(* Logix 5000 AddOnInstructionDefinition export HI6200_Faceplate_AOI; software revision 30.00 *)

ADD_ON_INSTRUCTION HI6200_Faceplate_AOI   (* revision 1.1, vendor Hardy Process Solutions *)
// AOI to run sample faceplate.
// Revision note:
// modified tag names to be more descriptive.
// Made code more efficient.
VAR_OUTPUT
   cal_status : SINT; {access Read Only}   // filtered cal status
END_VAR
VAR_INPUT
   fp_dis_md : INT;   // weight select
END_VAR
VAR_OUTPUT
   cmd_status : DINT; {access Read Only}   // filtered cmd status
END_VAR
VAR_IN_OUT
   Input_hi6200 : _0102:Hardy6200Series_F6857DC7:I:0; {required}
   Output_hi6200 : _0102:Hardy6200Series_52E4DDE0:O:0; {required}
END_VAR
VAR_INPUT
   pm_2881 : DINT;   // Units of measure
END_VAR
VAR_OUTPUT
   hardy_6200_inst_st : INT; {access Read Only}   // Instrument Status
   hardy_6200_net_wt : REAL; {access Read Only}   // Net Weight
   hardy_6200_gross_wt : REAL; {access Read Only}   // Gross weight
END_VAR
VAR_INPUT
   pm_4101 : REAL;   // Ref Weight
   pm_4182 : REAL;   // Span Weight
   pm_4102 : REAL;   // Gravity Correction
   pm_2081 : DINT;   // WAVERSAVER
   pm_2082 : DINT;   // Averages
   pm_6301 : DINT;   // Auto Zero Tracking Enable
   reset_az_enable_indication : BOOL;   // reset pointer on HMI list for Zero Tracking
   pm_6302 : REAL;   // Auto Zero tolerance
   pm_2886 : REAL;   // Zero Tolerance
END_VAR
VAR_OUTPUT
   pm_6201 : REAL;   // previous zerod amount
END_VAR
VAR_INPUT
   reset_units_indication : BOOL;   // reset pointer on HMI list for units of measure
   pm_2887 : REAL;   // Motion tolerance
   pm_6183 : REAL;   // Tare Weight
   reset_waversaver_indicator : BOOL;   // reset pointer on HMI list for WAVERSAVER
   rd_filter_settings : BOOL;   // Read filter settings
   input_cmd_status : INT;   // Filtered Cmd Status
   rd_zero_tare_settings : BOOL;   // read zero and tare settings
   rd_setup1_settings : BOOL;   // read setup 1 settings
   rd_c2cal_settings : BOOL;   // read C2 cal settings
   rd_tradcal_settings : BOOL;   // program control bit to read hard cal ref weight
   zero_cmd : BOOL;   // trigger zero command
   tare_cmd : BOOL;   // trigger tare command
   cal_low_cmd : BOOL;   // Cal Low trigger
   cal_high_cmd : BOOL;   // Cal High trigger
   c2_cmd : BOOL;   // C2 cal trigger
   write_C2_cal_settings : BOOL;   // trigger write C2 settings
   write_tradcal_settings : BOOL;   // trigger write hard cal settings
   write_filter_settings : BOOL;   // trigger write filter settings
   write_zero_tare_settings : BOOL;   // trigger write zero and tare settings
   write_units_setting : BOOL;   // trigger write units of measure
   pm_2888 : REAL;   // Capacity
   rd_setup2_settings : BOOL;   // read setup 2 settings
   pm_2882 : DINT;   // Decimal places
   pm_2883 : DINT;   // Grad size
   reset_decimalpoint_indication : BOOL;   // reset pointer on HMI list for decimal point
   reset_grads_indication : BOOL;   // reset pointer on HMI list for grad size
   pm_4081 : DINT;   // Sensitivity
   reset_sensitivity_indication : BOOL;   // reset pointer on HMI list for sensitivity
   write_setup2_settings : BOOL;   // trigger write ins settup 2 settings
   write_setup1_settings : BOOL;   // trigger write ins setup 1 settings
END_VAR
VAR_IN_OUT
   config_6200 : _0102:Hardy6200Series_ABC98FB2:C:0; {required}
END_VAR
VAR_INPUT
   percent_weight : REAL;   // percent of full scale for trend
   Set_FaceplateAnimation : INT;   // HMI panel control
   pm_2081w : DINT;   // write value setting for WAVERSAVER
   pm_6301w : DINT;   // write value setting for auto zero tracking enable
   pm_2881w : DINT;   // write value for setting units of measure
   pm_2882w : DINT;   // write value for setting decimal places
   pm_2883w : DINT;   // write value for setting grad size
   pm_4081w : DINT;   // write value for setting sensitivity value
END_VAR
VAR
   initial_unit_rd : BOOL; {access None}   // program control bit to initial read of units of measure
   cmd_no : INT; {access None}   // cmd num holding register
   ons_1 : BOOL; {access None}
   ons_2 : BOOL; {access None}
   rd_waversaver : BOOL; {access None}   // read WAVERSAVER setting
   delay_reset_waversaer_ind : TIMER := (PRE := 200); {access None}   // operational delay timer
   rd_az_zero_tol : BOOL; {access None}   // read auto zero tolerance
   delay_reset_az_enable_indication : TIMER := (PRE := 200); {access None}   // operational delay timer
   rd_zero_tol : BOOL; {access None}   // read zero tolerance
   rd_zero_amount : BOOL; {access None}   // read zero'd amount
   ons_3 : BOOL; {access None}
   rd_motion_tol : BOOL; {access None}   // program control for read motion tol
   rd_capacity : BOOL; {access None}   // program control for read capacity
   delay_reset_units_indication : TIMER := (PRE := 200); {access None}   // operational delay timer
   ons_4 : BOOL; {access None}
   rd_c2cal_ref_wt : BOOL; {access None}   // program control during read C2 cal ref weight
   ons_5 : BOOL; {access None}
   rd_tradcal_span_wt : BOOL; {access None}   // program control bit to read hard cal span weight
   ons_6 : BOOL; {access None}
   ons_7 : BOOL; {access None}
   ons_8 : BOOL; {access None}
   ons_9 : BOOL; {access None}
   ons_10 : BOOL; {access None}
   run_cmd : BOOL; {access None}   // program control bit
   run_cmd_delay : TIMER := (PRE := 1000); {access None}   // Delay timer to allow time for process to complete
   ons_11 : BOOL; {access None}
   wr_C2_ref_wt : BOOL; {access None}   // program control bit writing C2 ref weight
   chec_status_wr_C2_ref : BOOL; {access None}   // operational code control bit writing C2 ref
   wr_gravity_correction : BOOL; {access None}   // program control bit writing gravity correction
   check_status_wr_gravity_correction : BOOL; {access None}   // operational code control bit write gravity correction
   ons_12 : BOOL; {access None}
   wr_hard_cal_ref_wt : BOOL; {access None}   // program control bit writing hard cal ref weight
   check_status_wr_traditional_ref : BOOL; {access None}   // operational code control bit write hard cal ref
   wr_span_wt : BOOL; {access None}   // program control bit writing span weight
   check_status_wr_span_wt : BOOL; {access None}   // operational code control bit write span weight
   ons_13 : BOOL; {access None}
   wr_waversaver : BOOL; {access None}   // program control bit writing WAVERSAVER
   check_status_wr_waversaver : BOOL; {access None}   // operational code control bit write WAVERSAVER
   wr_avgerages : BOOL; {access None}   // program control bit writing averages
   check_status_wr_averages : BOOL; {access None}   // operational code control bit write Averages
   wr_auto_zero_enable : BOOL; {access None}   // program control bit writing zuto zero enable
   check_status_wr_auto_zero_enable : BOOL; {access None}   // operational code control bit writing Auto Zero enable
   ons_14 : BOOL; {access None}
   wr_auto_zero_tolerance : BOOL; {access None}   // program control bit writing auto zero tolerance
   check_status_wr_auto_zero_tolerance : BOOL; {access None}   // operational code control bit writing Auto Zero tolerance
   wr_zero_tolerance : BOOL; {access None}   // program control bit writing zero tolerance
   check_status_wr_zero_tolerance : BOOL; {access None}   // operational code control bit write zero tolerance
   wr_units_measure : BOOL; {access None}   // program control bit writing units of measure
   ons_15 : BOOL; {access None}
   check_status_wr_units_measure : BOOL; {access None}   // operational code control bit write units of measure
   wr_motion_tolerance : BOOL; {access None}   // program control bit writing motion tolerance
   check_status_wr_motion_tolerance : BOOL; {access None}   // operational code control bit write motion tolerance
   wr_tare_weight : BOOL; {access None}   // program control bit writing tare weight
   check_status_wr_tare_weight : BOOL; {access None}   // operational code control bit write tare weight
   rd_tare_weight : BOOL; {access None}   // read tare weight
   ons_16 : BOOL; {access None}
   rd_grad_size : BOOL; {access None}   // program control bit for read grad size
   delay_reset_decimalpoint_indication : TIMER := (PRE := 200); {access None}   // operational delay timer
   delay_reset_grads_indication : TIMER := (PRE := 200); {access None}   // operational delay timer
   rd_hardcal_sensitivity : BOOL; {access None}   // program control bit to read hard cal sensitivity
   delay_reset_sensitivity_indication : TIMER := (PRE := 200); {access None}   // operational delay timer
   wr_sensitivity : BOOL; {access None}   // program control bit writing sensitivity
   check_status_wr_sensitivity : BOOL; {access None}   // operational code control bit write sensitivity
   wr_scale_capacity : BOOL; {access None}   // program control bit writing scale capacity
   check_status_wr_scale_capacity : BOOL; {access None}   // operational code control bit write scale capacity
   ons_17 : BOOL; {access None}
   wr_decimal_point : BOOL; {access None}   // program control bit writing decimal point
   check_status_wr_decimal_point : BOOL; {access None}   // operational code control bit writing decimal points
   wr_grad_size : BOOL; {access None}   // program control bit writing grad size
   check_status_wr_grads_size : BOOL; {access None}   // operational code control bit write grad size
   ons_18 : BOOL; {access None}
   rd_averages : BOOL; {access None}   // program control tag to read averages
   rd_autozero_state : BOOL; {access None}   // program control bit to read auto zero tracking state
   rd_units_measure : BOOL; {access None}   // program control bit to read the units of measure
   rd_decimal_places : BOOL; {access None}   // program control bit to read decima places
   rd_gravity : BOOL; {access None}   // program control bit to read gravity correction
   rd_traditional_cal_ref_wt : BOOL; {access None}   // program control bit to read traditional cal ref weight
   initial_capacity_rd : BOOL; {access None}   // program control bit to initial read of scale capacity
   initial_unit_rd_1 : BOOL; {access None}   // program control bit
   delay_dec_rd : TIMER := (PRE := 300); {access None}   // delay timer for decimal pt read
   delay_units_rd : TIMER := (PRE := 200); {access None}   // delay timer for units read
   delay_zstate_rd : TIMER := (PRE := 200); {access None}   // delay timer for zero state read
   delay_wave_rd : TIMER := (PRE := 200); {access None}   // delay timer for waversaver read
END_VAR

ROUTINE Logic   (* ladder *)
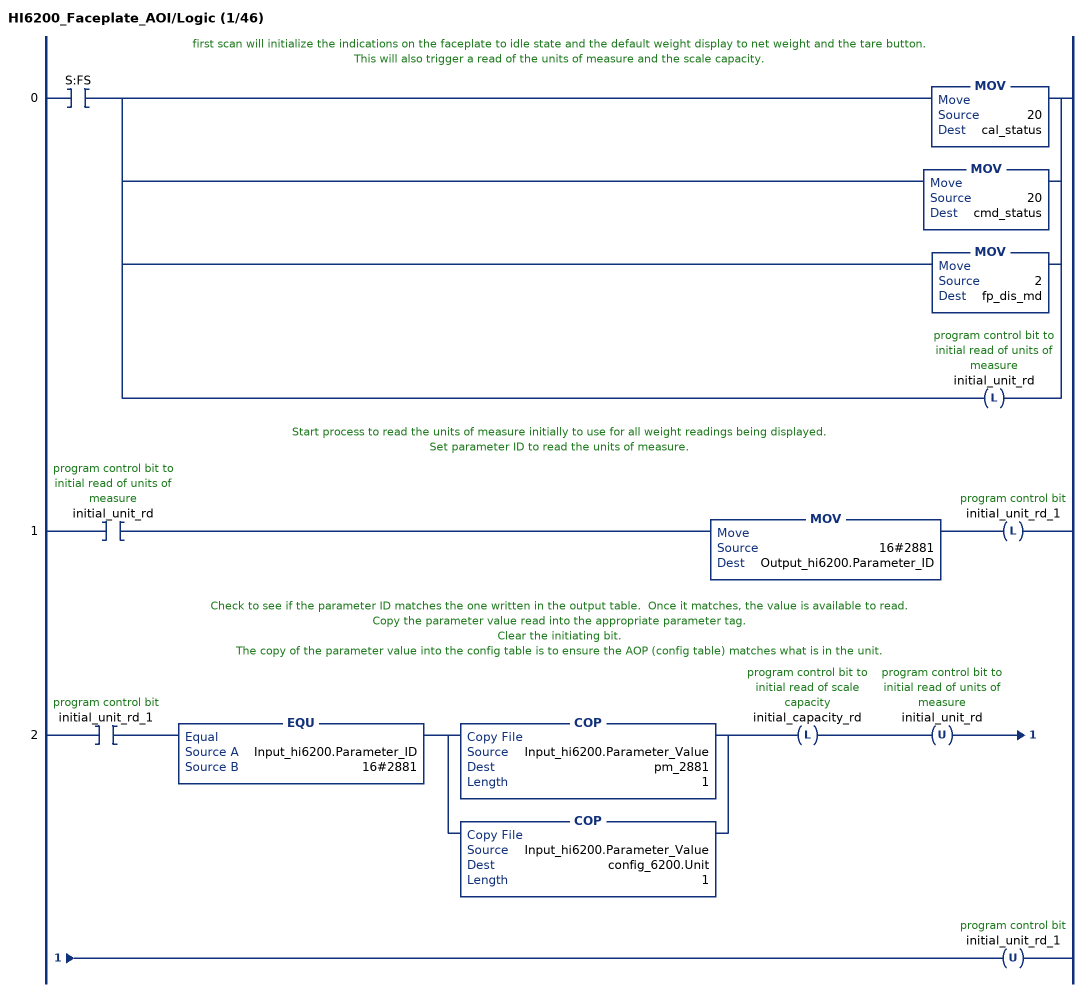
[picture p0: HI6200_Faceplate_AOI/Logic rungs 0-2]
   // first scan will initialize the indications on the faceplate to idle state and the default weight display to net weight and the tare button.
   // This will also trigger a read of the units of measure and the scale capacity.
   0: XIC(S:FS)[MOV(20,cal_status) ,MOV(20,cmd_status) ,MOV(2,fp_dis_md) ,OTL(initial_unit_rd) ];
   // Start process to read the units of measure initially to use for all weight readings being displayed.
   // Set parameter ID to read the units of measure.
   1: XIC(initial_unit_rd)MOV(16#2881,Output_hi6200.Parameter_ID)OTL(initial_unit_rd_1);
   // Check to see if the parameter ID matches the one written in the output table.  Once it matches, the value is available to read.
   // Copy the parameter value read into the appropriate parameter tag.
   // Clear the initiating bit.
   // The copy of the parameter value into the config table is to ensure the AOP (config table) matches what is in the unit.
   2: XIC(initial_unit_rd_1)EQU(Input_hi6200.Parameter_ID,16#2881)[COP(Input_hi6200.Parameter_Value,pm_2881,1) ,COP(Input_hi6200.Parameter_Value,config_6200.Unit,1) ]OTL(initial_capacity_rd)OTU(initial_unit_rd)OTU(initial_unit_rd_1);
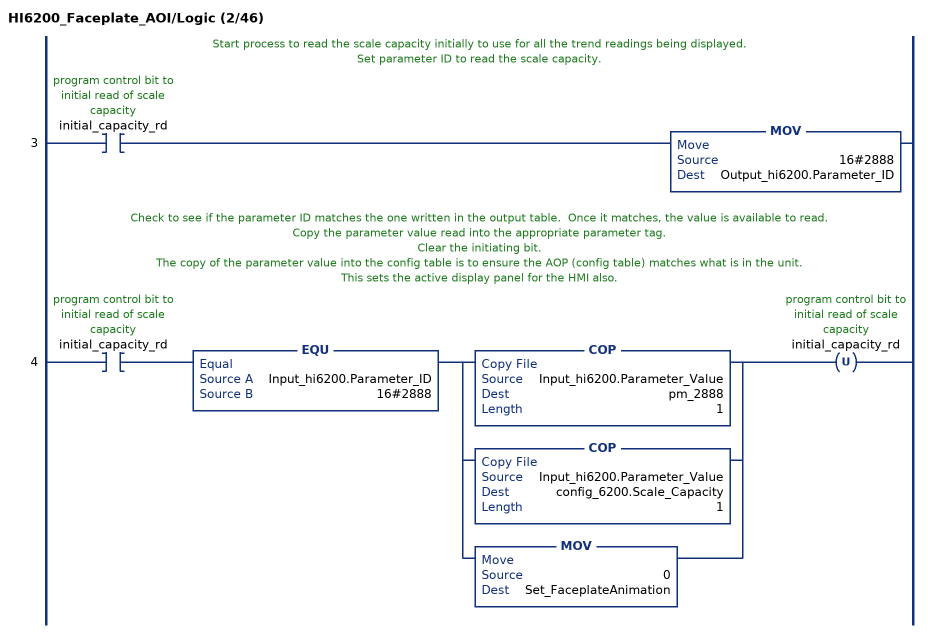
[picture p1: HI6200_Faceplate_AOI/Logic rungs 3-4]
   // Start process to read the scale capacity initially to use for all the trend readings being displayed.
   // Set parameter ID to read the scale capacity.
   3: XIC(initial_capacity_rd)MOV(16#2888,Output_hi6200.Parameter_ID);
   // Check to see if the parameter ID matches the one written in the output table.  Once it matches, the value is available to read.
   // Copy the parameter value read into the appropriate parameter tag.
   // Clear the initiating bit.
   // The copy of the parameter value into the config table is to ensure the AOP (config table) matches what is in the unit.
   // This sets the active display panel for the HMI also.
   4: XIC(initial_capacity_rd)EQU(Input_hi6200.Parameter_ID,16#2888)[COP(Input_hi6200.Parameter_Value,pm_2888,1) ,COP(Input_hi6200.Parameter_Value,config_6200.Scale_Capacity,1) ,MOV(0,Set_FaceplateAnimation) ]OTU(initial_capacity_rd);
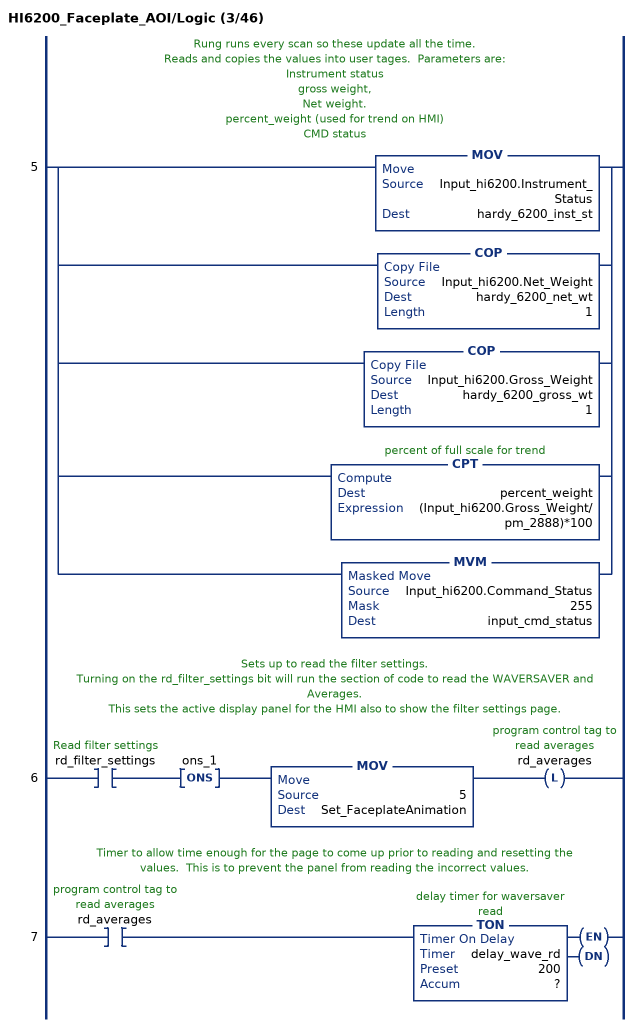
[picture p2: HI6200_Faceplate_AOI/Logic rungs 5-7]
   // Rung runs every scan so these update all the time.
   // Reads and copies the values into user tages.  Parameters are:
   // Instrument status
   // gross weight,
   // Net weight.
   // percent_weight (used for trend on HMI)
   // CMD status
   5: [MOV(Input_hi6200.Instrument_Status,hardy_6200_inst_st) ,COP(Input_hi6200.Net_Weight,hardy_6200_net_wt,1) ,COP(Input_hi6200.Gross_Weight,hardy_6200_gross_wt,1) ,CPT(percent_weight,(Input_hi6200.Gross_Weight/pm_2888)*100) ,MVM(Input_hi6200.Command_Status,255,input_cmd_status) ];
   // Sets up to read the filter settings.
   // Turning on the rd_filter_settings bit will run the section of code to read the WAVERSAVER and Averages.
   // This sets the active display panel for the HMI also to show the filter settings page.
   6: XIC(rd_filter_settings)ONS(ons_1)MOV(5,Set_FaceplateAnimation)OTL(rd_averages);
   // Timer to allow time enough for the page to come up prior to reading and resetting the values.  This is to prevent the panel from reading the incorrect values.
   7: XIC(rd_averages)TON(delay_wave_rd,?,?);
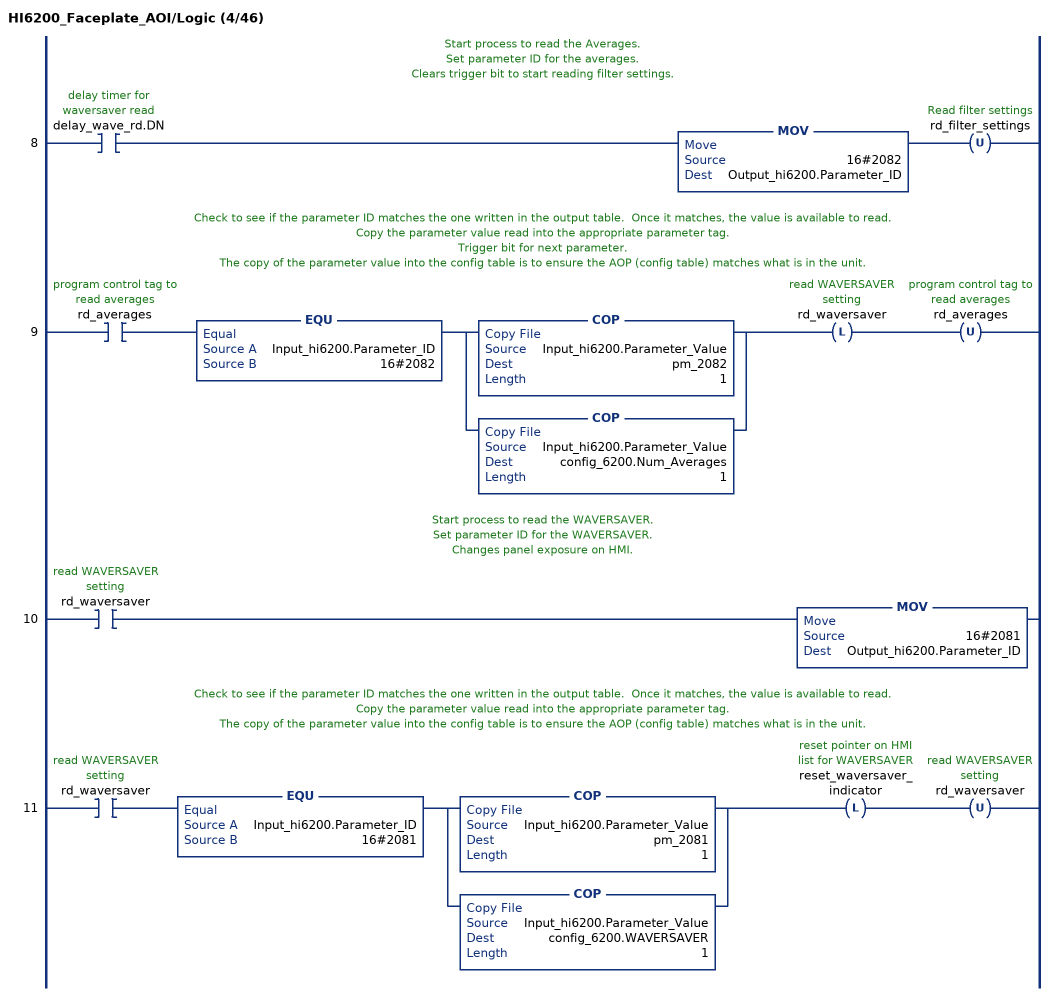
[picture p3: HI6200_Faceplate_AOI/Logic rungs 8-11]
   // Start process to read the Averages.
   // Set parameter ID for the averages.
   // Clears trigger bit to start reading filter settings.
   8: XIC(delay_wave_rd.DN)MOV(16#2082,Output_hi6200.Parameter_ID)OTU(rd_filter_settings);
   // Check to see if the parameter ID matches the one written in the output table.  Once it matches, the value is available to read.
   // Copy the parameter value read into the appropriate parameter tag.
   // Trigger bit for next parameter.
   // The copy of the parameter value into the config table is to ensure the AOP (config table) matches what is in the unit.
   9: XIC(rd_averages)EQU(Input_hi6200.Parameter_ID,16#2082)[COP(Input_hi6200.Parameter_Value,pm_2082,1) ,COP(Input_hi6200.Parameter_Value,config_6200.Num_Averages,1) ]OTL(rd_waversaver)OTU(rd_averages);
   // Start process to read the WAVERSAVER.
   // Set parameter ID for the WAVERSAVER.
   // Changes panel exposure on HMI.
   10: XIC(rd_waversaver)MOV(16#2081,Output_hi6200.Parameter_ID);
   // Check to see if the parameter ID matches the one written in the output table.  Once it matches, the value is available to read.
   // Copy the parameter value read into the appropriate parameter tag.
   // The copy of the parameter value into the config table is to ensure the AOP (config table) matches what is in the unit.
   11: XIC(rd_waversaver)EQU(Input_hi6200.Parameter_ID,16#2081)[COP(Input_hi6200.Parameter_Value,pm_2081,1) ,COP(Input_hi6200.Parameter_Value,config_6200.WAVERSAVER,1) ]OTL(reset_waversaver_indicator)OTU(rd_waversaver);
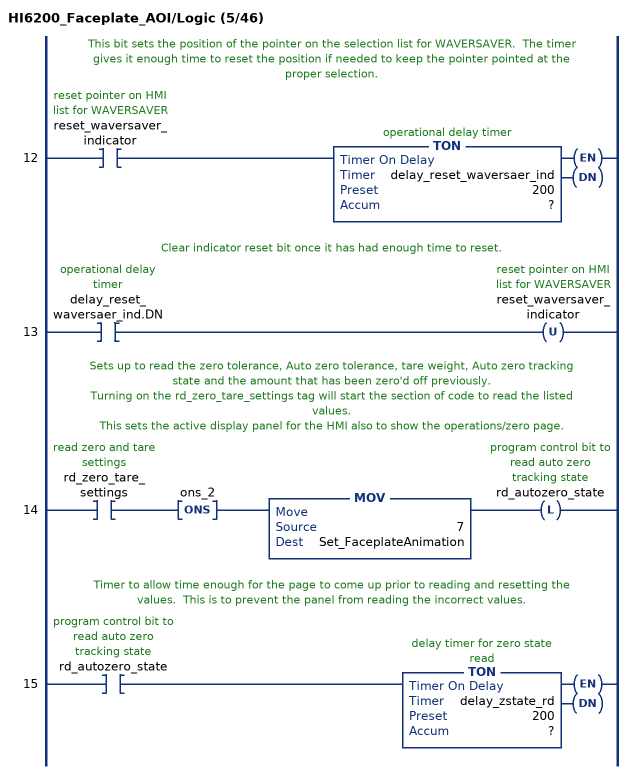
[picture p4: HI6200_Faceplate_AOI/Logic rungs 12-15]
   // This bit sets the position of the pointer on the selection list for WAVERSAVER.  The timer gives it enough time to reset the position if needed to keep the pointer pointed at the proper selection.
   12: XIC(reset_waversaver_indicator)TON(delay_reset_waversaer_ind,?,?);
   // Clear indicator reset bit once it has had enough time to reset.
   13: XIC(delay_reset_waversaer_ind.DN)OTU(reset_waversaver_indicator);
   // Sets up to read the zero tolerance, Auto zero tolerance, tare weight, Auto zero tracking state and the amount that has been zero'd off previously.
   // Turning on the rd_zero_tare_settings tag will start the section of code to read the listed values.
   // This sets the active display panel for the HMI also to show the operations/zero page.
   14: XIC(rd_zero_tare_settings)ONS(ons_2)MOV(7,Set_FaceplateAnimation)OTL(rd_autozero_state);
   // Timer to allow time enough for the page to come up prior to reading and resetting the values.  This is to prevent the panel from reading the incorrect values.
   15: XIC(rd_autozero_state)TON(delay_zstate_rd,?,?);
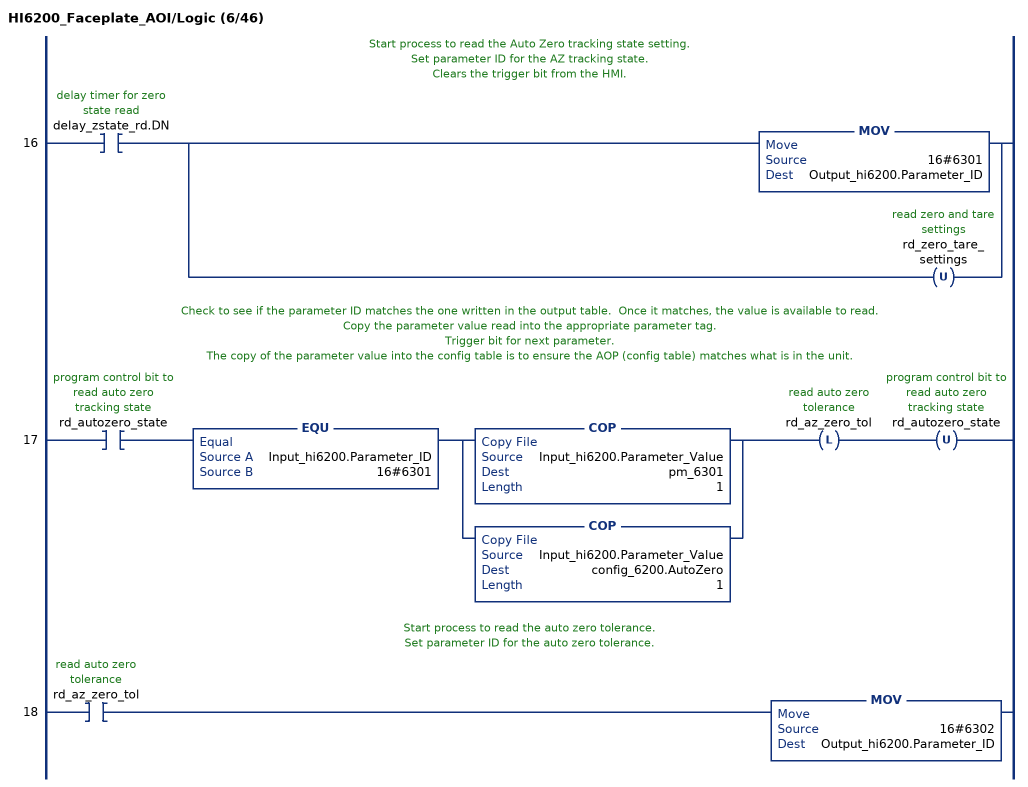
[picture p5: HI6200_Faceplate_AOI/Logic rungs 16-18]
   // Start process to read the Auto Zero tracking state setting.
   // Set parameter ID for the AZ tracking state.
   // Clears the trigger bit from the HMI.
   16: XIC(delay_zstate_rd.DN)[MOV(16#6301,Output_hi6200.Parameter_ID) ,OTU(rd_zero_tare_settings) ];
   // Check to see if the parameter ID matches the one written in the output table.  Once it matches, the value is available to read.
   // Copy the parameter value read into the appropriate parameter tag.
   // Trigger bit for next parameter.
   // The copy of the parameter value into the config table is to ensure the AOP (config table) matches what is in the unit.
   17: XIC(rd_autozero_state)EQU(Input_hi6200.Parameter_ID,16#6301)[COP(Input_hi6200.Parameter_Value,pm_6301,1) ,COP(Input_hi6200.Parameter_Value,config_6200.AutoZero,1) ]OTL(rd_az_zero_tol)OTU(rd_autozero_state);
   // Start process to read the auto zero tolerance.
   // Set parameter ID for the auto zero tolerance.
   18: XIC(rd_az_zero_tol)MOV(16#6302,Output_hi6200.Parameter_ID);
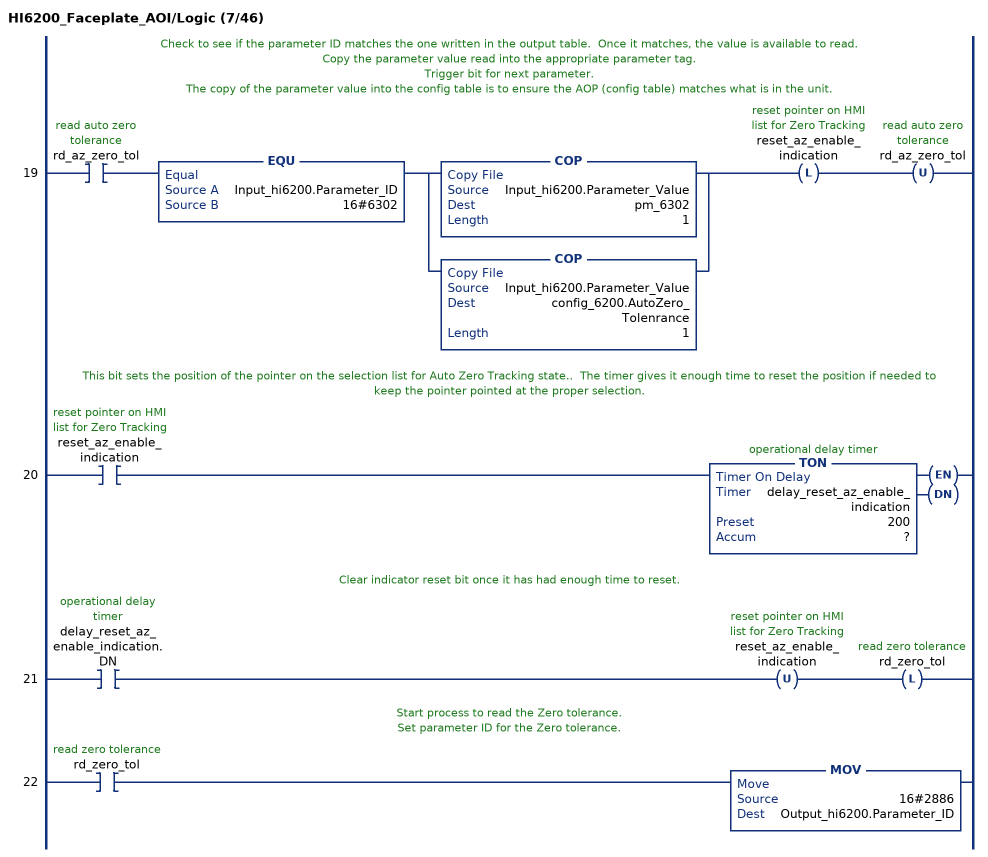
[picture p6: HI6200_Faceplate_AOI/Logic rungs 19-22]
   // Check to see if the parameter ID matches the one written in the output table.  Once it matches, the value is available to read.
   // Copy the parameter value read into the appropriate parameter tag.
   // Trigger bit for next parameter.
   // The copy of the parameter value into the config table is to ensure the AOP (config table) matches what is in the unit.
   19: XIC(rd_az_zero_tol)EQU(Input_hi6200.Parameter_ID,16#6302)[COP(Input_hi6200.Parameter_Value,pm_6302,1) ,COP(Input_hi6200.Parameter_Value,config_6200.AutoZero_Tolenrance,1) ]OTL(reset_az_enable_indication)OTU(rd_az_zero_tol);
   // This bit sets the position of the pointer on the selection list for Auto Zero Tracking state..  The timer gives it enough time to reset the position if needed to keep the pointer pointed at the proper selection.
   20: XIC(reset_az_enable_indication)TON(delay_reset_az_enable_indication,?,?);
   // Clear indicator reset bit once it has had enough time to reset.
   21: XIC(delay_reset_az_enable_indication.DN)OTU(reset_az_enable_indication)OTL(rd_zero_tol);
   // Start process to read the Zero tolerance.
   // Set parameter ID for the Zero tolerance.
   22: XIC(rd_zero_tol)MOV(16#2886,Output_hi6200.Parameter_ID);
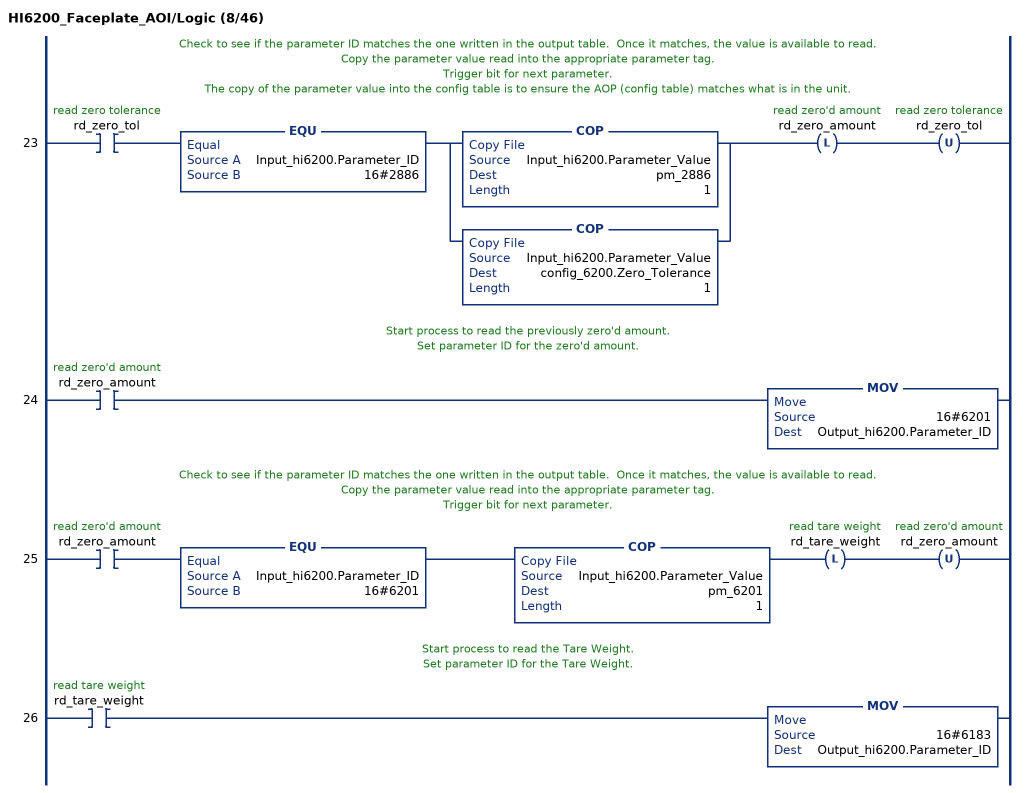
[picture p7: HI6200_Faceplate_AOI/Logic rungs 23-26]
   // Check to see if the parameter ID matches the one written in the output table.  Once it matches, the value is available to read.
   // Copy the parameter value read into the appropriate parameter tag.
   // Trigger bit for next parameter.
   // The copy of the parameter value into the config table is to ensure the AOP (config table) matches what is in the unit.
   23: XIC(rd_zero_tol)EQU(Input_hi6200.Parameter_ID,16#2886)[COP(Input_hi6200.Parameter_Value,pm_2886,1) ,COP(Input_hi6200.Parameter_Value,config_6200.Zero_Tolerance,1) ]OTL(rd_zero_amount)OTU(rd_zero_tol);
   // Start process to read the previously zero'd amount.
   // Set parameter ID for the zero'd amount.
   24: XIC(rd_zero_amount)MOV(16#6201,Output_hi6200.Parameter_ID);
   // Check to see if the parameter ID matches the one written in the output table.  Once it matches, the value is available to read.
   // Copy the parameter value read into the appropriate parameter tag.
   // Trigger bit for next parameter.
   25: XIC(rd_zero_amount)EQU(Input_hi6200.Parameter_ID,16#6201)COP(Input_hi6200.Parameter_Value,pm_6201,1)OTL(rd_tare_weight)OTU(rd_zero_amount);
   // Start process to read the Tare Weight.
   // Set parameter ID for the Tare Weight.
   26: XIC(rd_tare_weight)MOV(16#6183,Output_hi6200.Parameter_ID);
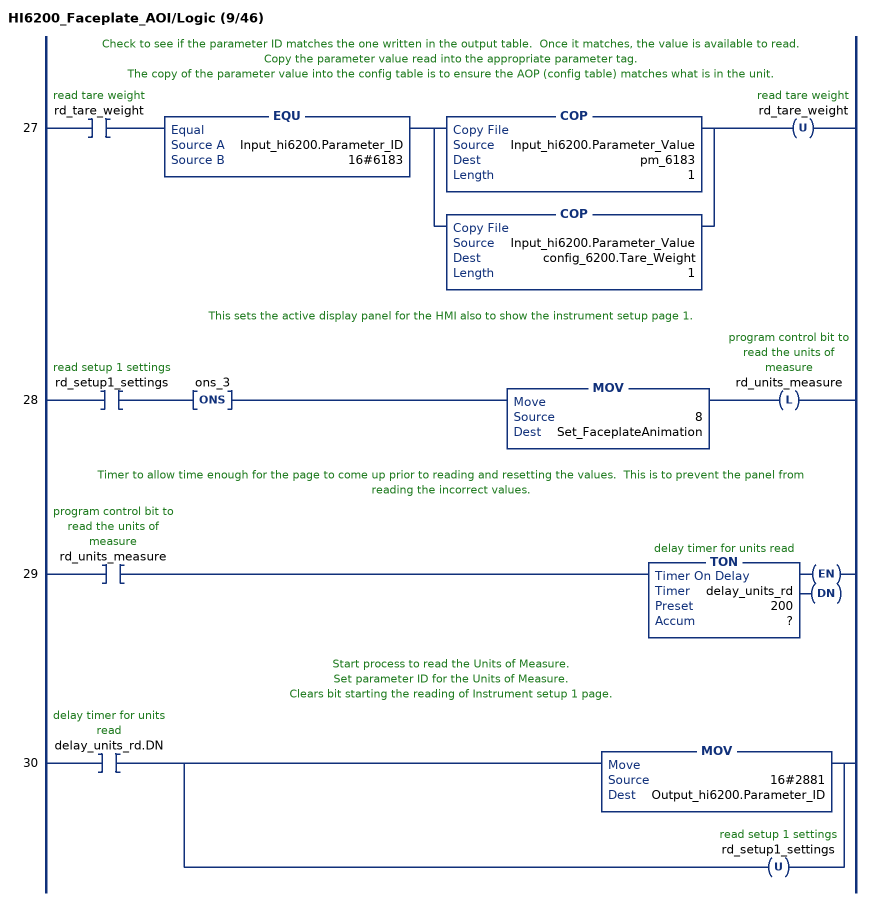
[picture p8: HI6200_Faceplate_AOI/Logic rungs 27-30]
   // Check to see if the parameter ID matches the one written in the output table.  Once it matches, the value is available to read.
   // Copy the parameter value read into the appropriate parameter tag.
   // The copy of the parameter value into the config table is to ensure the AOP (config table) matches what is in the unit.
   27: XIC(rd_tare_weight)EQU(Input_hi6200.Parameter_ID,16#6183)[COP(Input_hi6200.Parameter_Value,pm_6183,1) ,COP(Input_hi6200.Parameter_Value,config_6200.Tare_Weight,1) ]OTU(rd_tare_weight);
   // This sets the active display panel for the HMI also to show the instrument setup page 1.
   28: XIC(rd_setup1_settings)ONS(ons_3)MOV(8,Set_FaceplateAnimation)OTL(rd_units_measure);
   // Timer to allow time enough for the page to come up prior to reading and resetting the values.  This is to prevent the panel from reading the incorrect values.
   29: XIC(rd_units_measure)TON(delay_units_rd,?,?);
   // Start process to read the Units of Measure.
   // Set parameter ID for the Units of Measure.
   // Clears bit starting the reading of Instrument setup 1 page.
   30: XIC(delay_units_rd.DN)[MOV(16#2881,Output_hi6200.Parameter_ID) ,OTU(rd_setup1_settings) ];
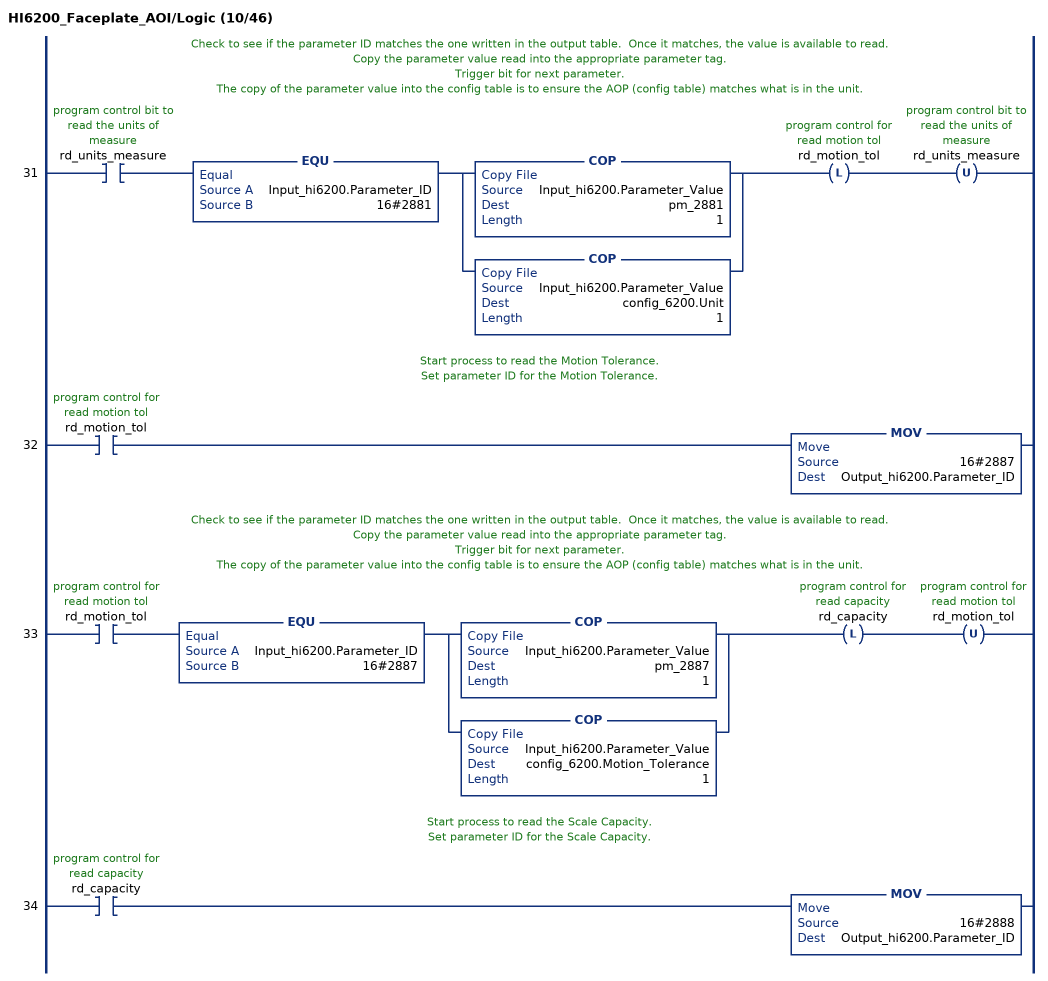
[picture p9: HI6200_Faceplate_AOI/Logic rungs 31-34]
   // Check to see if the parameter ID matches the one written in the output table.  Once it matches, the value is available to read.
   // Copy the parameter value read into the appropriate parameter tag.
   // Trigger bit for next parameter.
   // The copy of the parameter value into the config table is to ensure the AOP (config table) matches what is in the unit.
   31: XIC(rd_units_measure)EQU(Input_hi6200.Parameter_ID,16#2881)[COP(Input_hi6200.Parameter_Value,pm_2881,1) ,COP(Input_hi6200.Parameter_Value,config_6200.Unit,1) ]OTL(rd_motion_tol)OTU(rd_units_measure);
   // Start process to read the Motion Tolerance.
   // Set parameter ID for the Motion Tolerance.
   32: XIC(rd_motion_tol)MOV(16#2887,Output_hi6200.Parameter_ID);
   // Check to see if the parameter ID matches the one written in the output table.  Once it matches, the value is available to read.
   // Copy the parameter value read into the appropriate parameter tag.
   // Trigger bit for next parameter.
   // The copy of the parameter value into the config table is to ensure the AOP (config table) matches what is in the unit.
   33: XIC(rd_motion_tol)EQU(Input_hi6200.Parameter_ID,16#2887)[COP(Input_hi6200.Parameter_Value,pm_2887,1) ,COP(Input_hi6200.Parameter_Value,config_6200.Motion_Tolerance,1) ]OTL(rd_capacity)OTU(rd_motion_tol);
   // Start process to read the Scale Capacity.
   // Set parameter ID for the Scale Capacity.
   34: XIC(rd_capacity)MOV(16#2888,Output_hi6200.Parameter_ID);
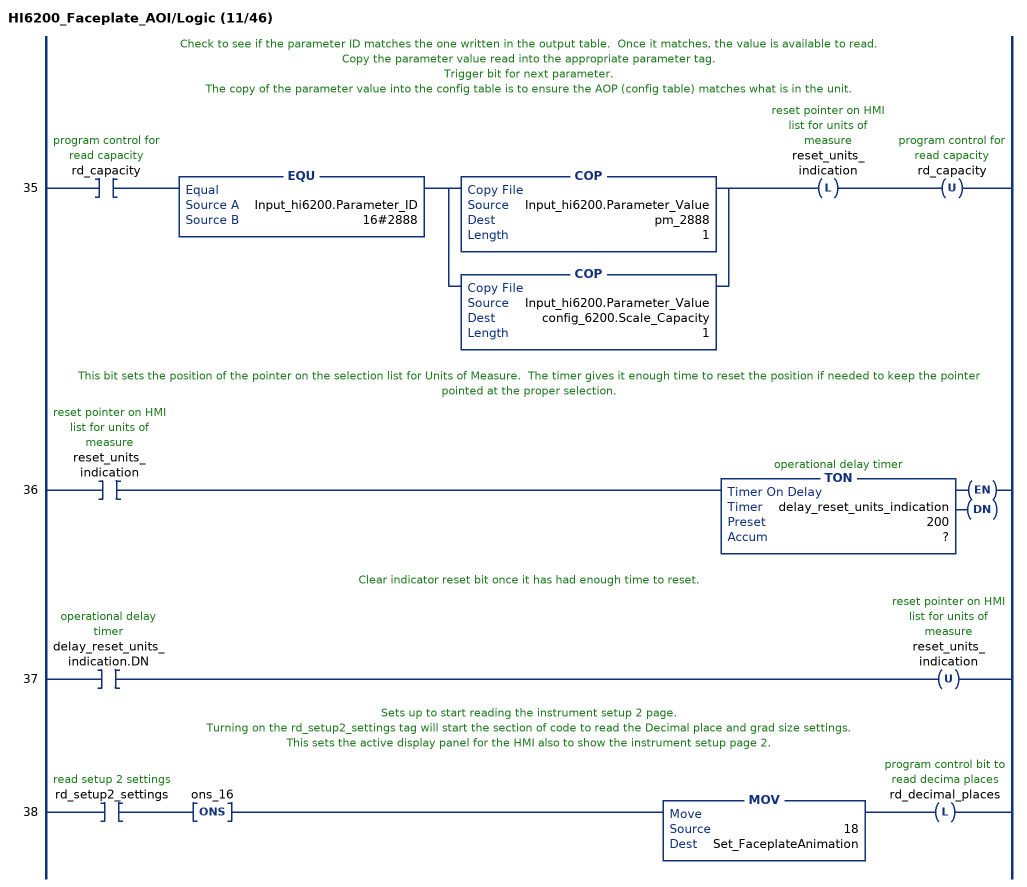
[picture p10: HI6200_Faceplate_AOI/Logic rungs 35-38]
   // Check to see if the parameter ID matches the one written in the output table.  Once it matches, the value is available to read.
   // Copy the parameter value read into the appropriate parameter tag.
   // Trigger bit for next parameter.
   // The copy of the parameter value into the config table is to ensure the AOP (config table) matches what is in the unit.
   35: XIC(rd_capacity)EQU(Input_hi6200.Parameter_ID,16#2888)[COP(Input_hi6200.Parameter_Value,pm_2888,1) ,COP(Input_hi6200.Parameter_Value,config_6200.Scale_Capacity,1) ]OTL(reset_units_indication)OTU(rd_capacity);
   // This bit sets the position of the pointer on the selection list for Units of Measure.  The timer gives it enough time to reset the position if needed to keep the pointer pointed at the proper selection.
   36: XIC(reset_units_indication)TON(delay_reset_units_indication,?,?);
   // Clear indicator reset bit once it has had enough time to reset.
   37: XIC(delay_reset_units_indication.DN)OTU(reset_units_indication);
   // Sets up to start reading the instrument setup 2 page.
   // Turning on the rd_setup2_settings tag will start the section of code to read the Decimal place and grad size settings.
   // This sets the active display panel for the HMI also to show the instrument setup page 2.
   38: XIC(rd_setup2_settings)ONS(ons_16)MOV(18,Set_FaceplateAnimation)OTL(rd_decimal_places);
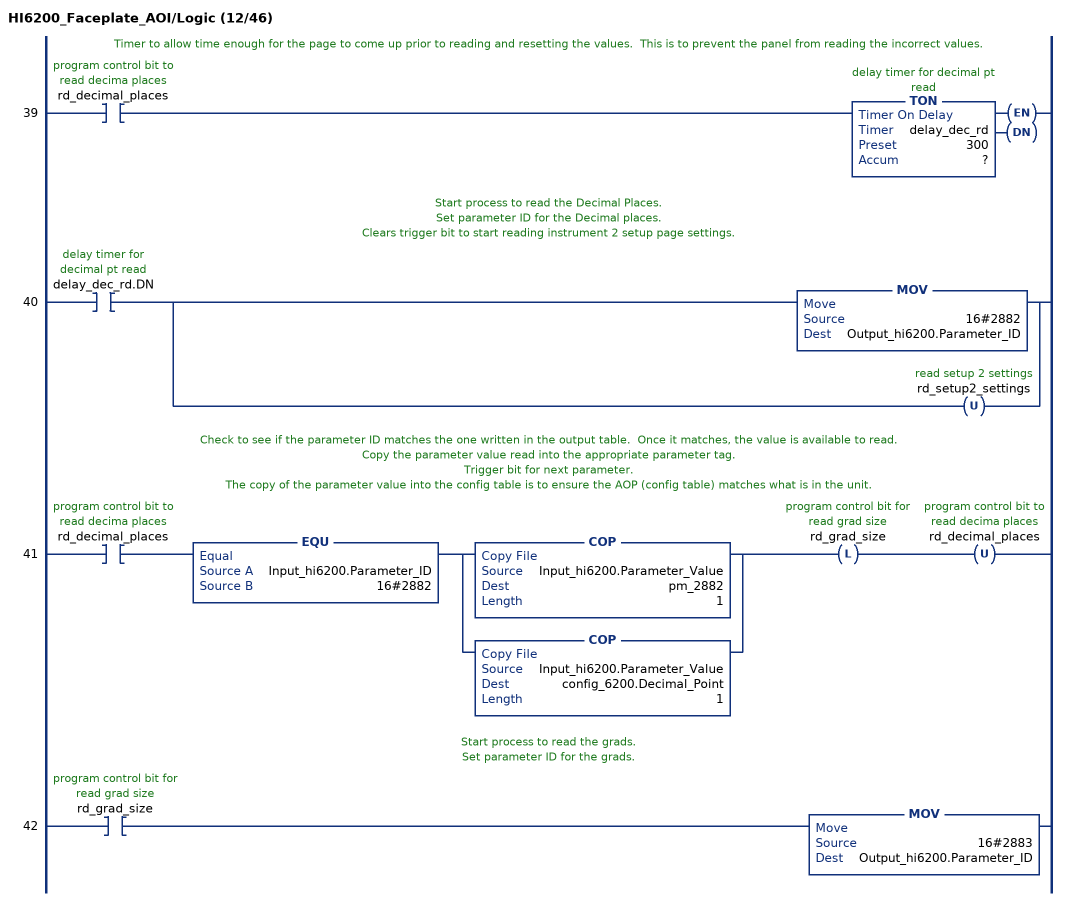
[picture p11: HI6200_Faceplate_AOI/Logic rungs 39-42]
   // Timer to allow time enough for the page to come up prior to reading and resetting the values.  This is to prevent the panel from reading the incorrect values.
   39: XIC(rd_decimal_places)TON(delay_dec_rd,?,?);
   // Start process to read the Decimal Places.
   // Set parameter ID for the Decimal places.
   // Clears trigger bit to start reading instrument 2 setup page settings.
   40: XIC(delay_dec_rd.DN)[MOV(16#2882,Output_hi6200.Parameter_ID) ,OTU(rd_setup2_settings) ];
   // Check to see if the parameter ID matches the one written in the output table.  Once it matches, the value is available to read.
   // Copy the parameter value read into the appropriate parameter tag.
   // Trigger bit for next parameter.
   // The copy of the parameter value into the config table is to ensure the AOP (config table) matches what is in the unit.
   41: XIC(rd_decimal_places)EQU(Input_hi6200.Parameter_ID,16#2882)[COP(Input_hi6200.Parameter_Value,pm_2882,1) ,COP(Input_hi6200.Parameter_Value,config_6200.Decimal_Point,1) ]OTL(rd_grad_size)OTU(rd_decimal_places);
   // Start process to read the grads.
   // Set parameter ID for the grads.
   42: XIC(rd_grad_size)MOV(16#2883,Output_hi6200.Parameter_ID);
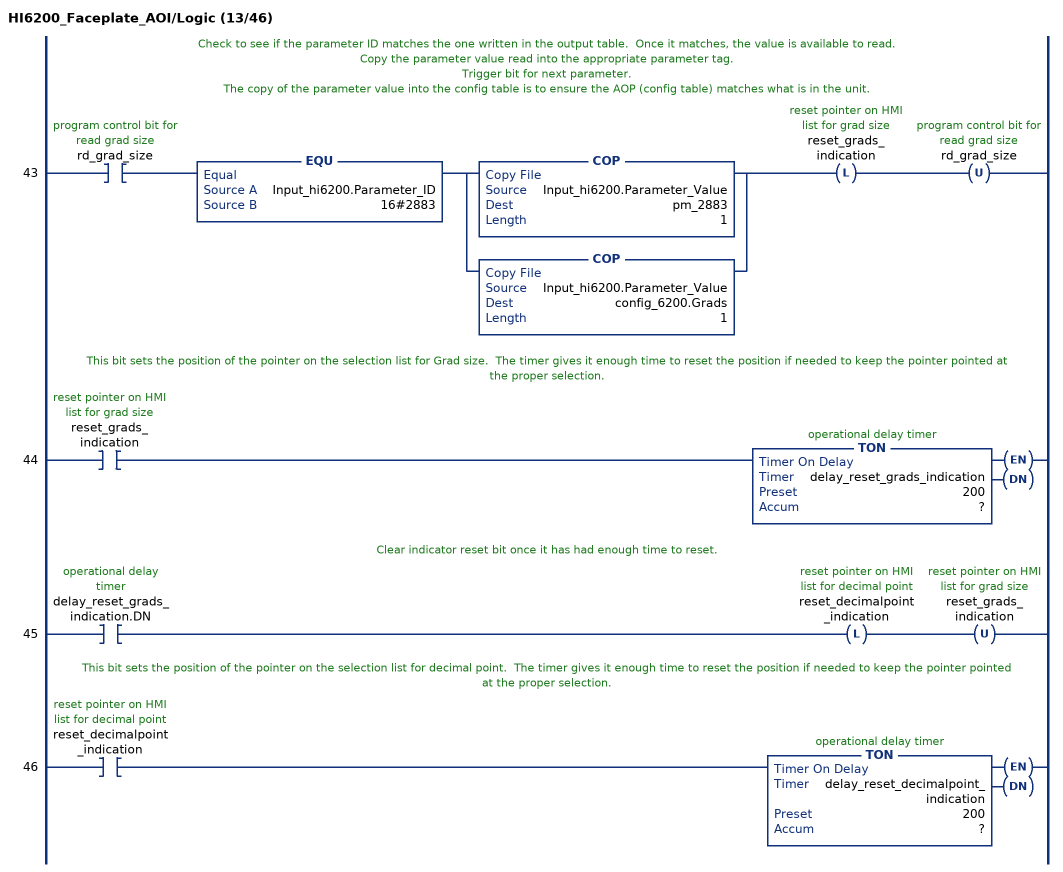
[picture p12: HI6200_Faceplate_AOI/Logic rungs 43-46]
   // Check to see if the parameter ID matches the one written in the output table.  Once it matches, the value is available to read.
   // Copy the parameter value read into the appropriate parameter tag.
   // Trigger bit for next parameter.
   // The copy of the parameter value into the config table is to ensure the AOP (config table) matches what is in the unit.
   43: XIC(rd_grad_size)EQU(Input_hi6200.Parameter_ID,16#2883)[COP(Input_hi6200.Parameter_Value,pm_2883,1) ,COP(Input_hi6200.Parameter_Value,config_6200.Grads,1) ]OTL(reset_grads_indication)OTU(rd_grad_size);
   // This bit sets the position of the pointer on the selection list for Grad size.  The timer gives it enough time to reset the position if needed to keep the pointer pointed at the proper selection.
   44: XIC(reset_grads_indication)TON(delay_reset_grads_indication,?,?);
   // Clear indicator reset bit once it has had enough time to reset.
   45: XIC(delay_reset_grads_indication.DN)OTL(reset_decimalpoint_indication)OTU(reset_grads_indication);
   // This bit sets the position of the pointer on the selection list for decimal point.  The timer gives it enough time to reset the position if needed to keep the pointer pointed at the proper selection.
   46: XIC(reset_decimalpoint_indication)TON(delay_reset_decimalpoint_indication,?,?);
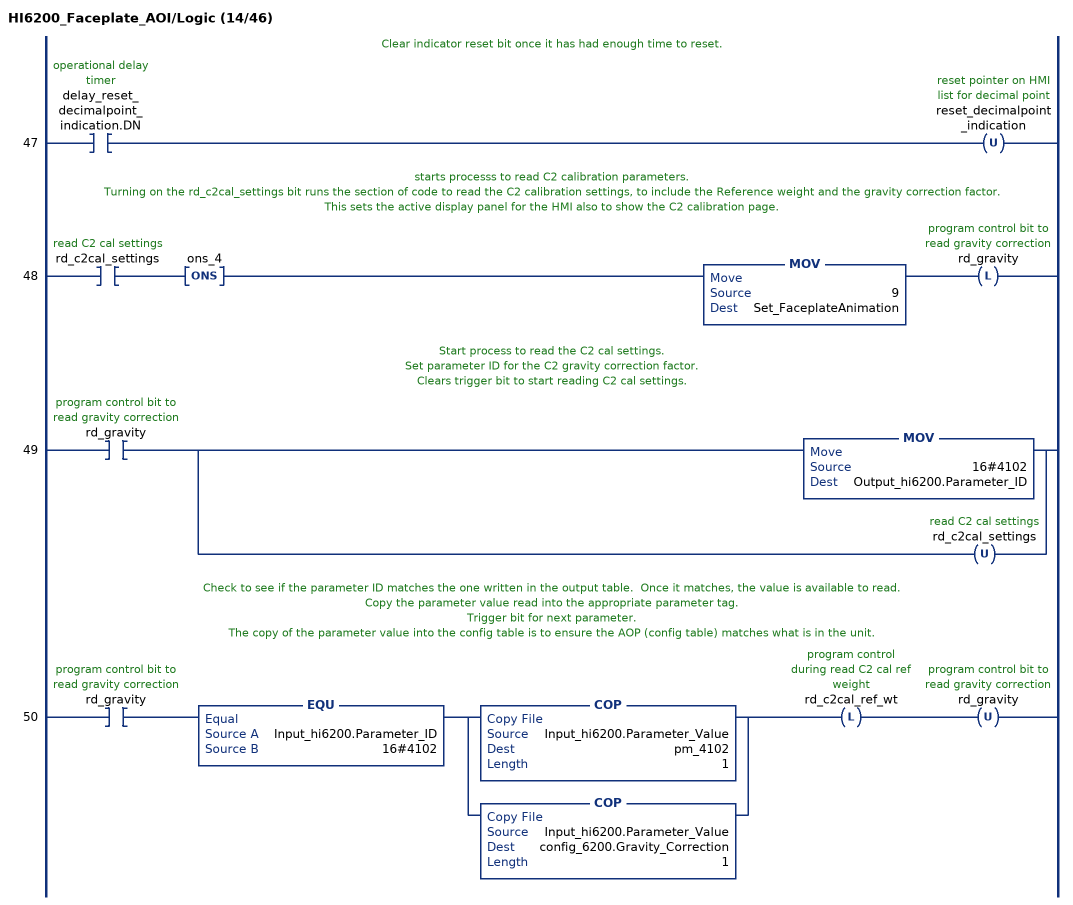
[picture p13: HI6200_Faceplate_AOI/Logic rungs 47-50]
   // Clear indicator reset bit once it has had enough time to reset.
   47: XIC(delay_reset_decimalpoint_indication.DN)OTU(reset_decimalpoint_indication);
   // starts processs to read C2 calibration parameters.
   // Turning on the rd_c2cal_settings bit runs the section of code to read the C2 calibration settings, to include the Reference weight and the gravity correction factor.
   // This sets the active display panel for the HMI also to show the C2 calibration page.
   48: XIC(rd_c2cal_settings)ONS(ons_4)MOV(9,Set_FaceplateAnimation)OTL(rd_gravity);
   // Start process to read the C2 cal settings.
   // Set parameter ID for the C2 gravity correction factor.
   // Clears trigger bit to start reading C2 cal settings.
   49: XIC(rd_gravity)[MOV(16#4102,Output_hi6200.Parameter_ID) ,OTU(rd_c2cal_settings) ];
   // Check to see if the parameter ID matches the one written in the output table.  Once it matches, the value is available to read.
   // Copy the parameter value read into the appropriate parameter tag.
   // Trigger bit for next parameter.
   // The copy of the parameter value into the config table is to ensure the AOP (config table) matches what is in the unit.
   50: XIC(rd_gravity)EQU(Input_hi6200.Parameter_ID,16#4102)[COP(Input_hi6200.Parameter_Value,pm_4102,1) ,COP(Input_hi6200.Parameter_Value,config_6200.Gravity_Correction,1) ]OTL(rd_c2cal_ref_wt)OTU(rd_gravity);
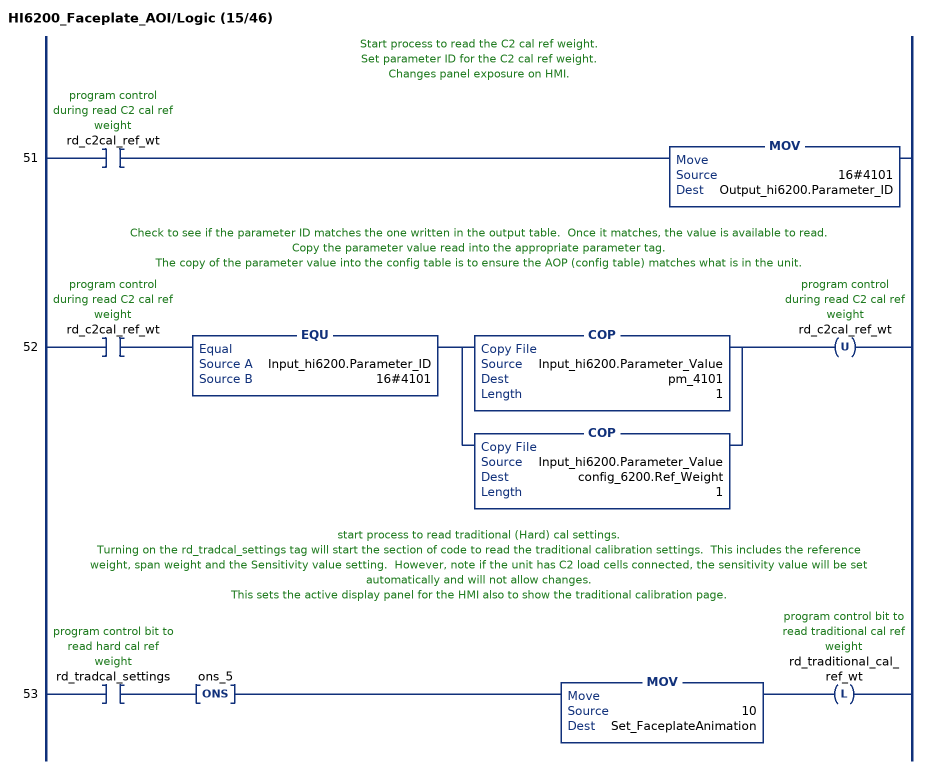
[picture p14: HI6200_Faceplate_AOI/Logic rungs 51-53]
   // Start process to read the C2 cal ref weight.
   // Set parameter ID for the C2 cal ref weight.
   // Changes panel exposure on HMI.
   51: XIC(rd_c2cal_ref_wt)MOV(16#4101,Output_hi6200.Parameter_ID);
   // Check to see if the parameter ID matches the one written in the output table.  Once it matches, the value is available to read.
   // Copy the parameter value read into the appropriate parameter tag.
   // The copy of the parameter value into the config table is to ensure the AOP (config table) matches what is in the unit.
   52: XIC(rd_c2cal_ref_wt)EQU(Input_hi6200.Parameter_ID,16#4101)[COP(Input_hi6200.Parameter_Value,pm_4101,1) ,COP(Input_hi6200.Parameter_Value,config_6200.Ref_Weight,1) ]OTU(rd_c2cal_ref_wt);
   // start process to read traditional (Hard) cal settings.
   // Turning on the rd_tradcal_settings tag will start the section of code to read the traditional calibration settings.  This includes the reference weight, span weight and the Sensitivity value setting.  However, note if the unit has C2 load cells connected, the sensitivity value will be set automatically and will not allow changes.
   // This sets the active display panel for the HMI also to show the traditional calibration page.
   53: XIC(rd_tradcal_settings)ONS(ons_5)MOV(10,Set_FaceplateAnimation)OTL(rd_traditional_cal_ref_wt);
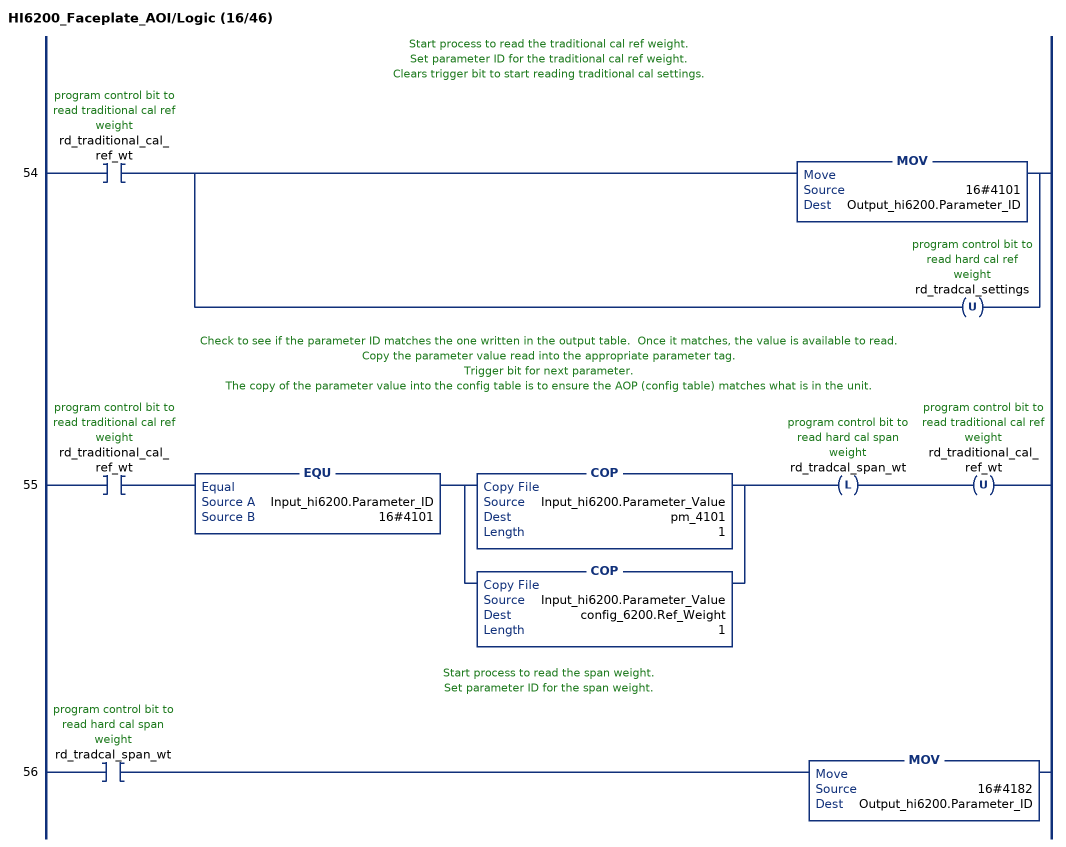
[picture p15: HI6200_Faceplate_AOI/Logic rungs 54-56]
   // Start process to read the traditional cal ref weight.
   // Set parameter ID for the traditional cal ref weight.
   // Clears trigger bit to start reading traditional cal settings.
   54: XIC(rd_traditional_cal_ref_wt)[MOV(16#4101,Output_hi6200.Parameter_ID) ,OTU(rd_tradcal_settings) ];
   // Check to see if the parameter ID matches the one written in the output table.  Once it matches, the value is available to read.
   // Copy the parameter value read into the appropriate parameter tag.
   // Trigger bit for next parameter.
   // The copy of the parameter value into the config table is to ensure the AOP (config table) matches what is in the unit.
   55: XIC(rd_traditional_cal_ref_wt)EQU(Input_hi6200.Parameter_ID,16#4101)[COP(Input_hi6200.Parameter_Value,pm_4101,1) ,COP(Input_hi6200.Parameter_Value,config_6200.Ref_Weight,1) ]OTL(rd_tradcal_span_wt)OTU(rd_traditional_cal_ref_wt);
   // Start process to read the span weight.
   // Set parameter ID for the span weight.
   56: XIC(rd_tradcal_span_wt)MOV(16#4182,Output_hi6200.Parameter_ID);
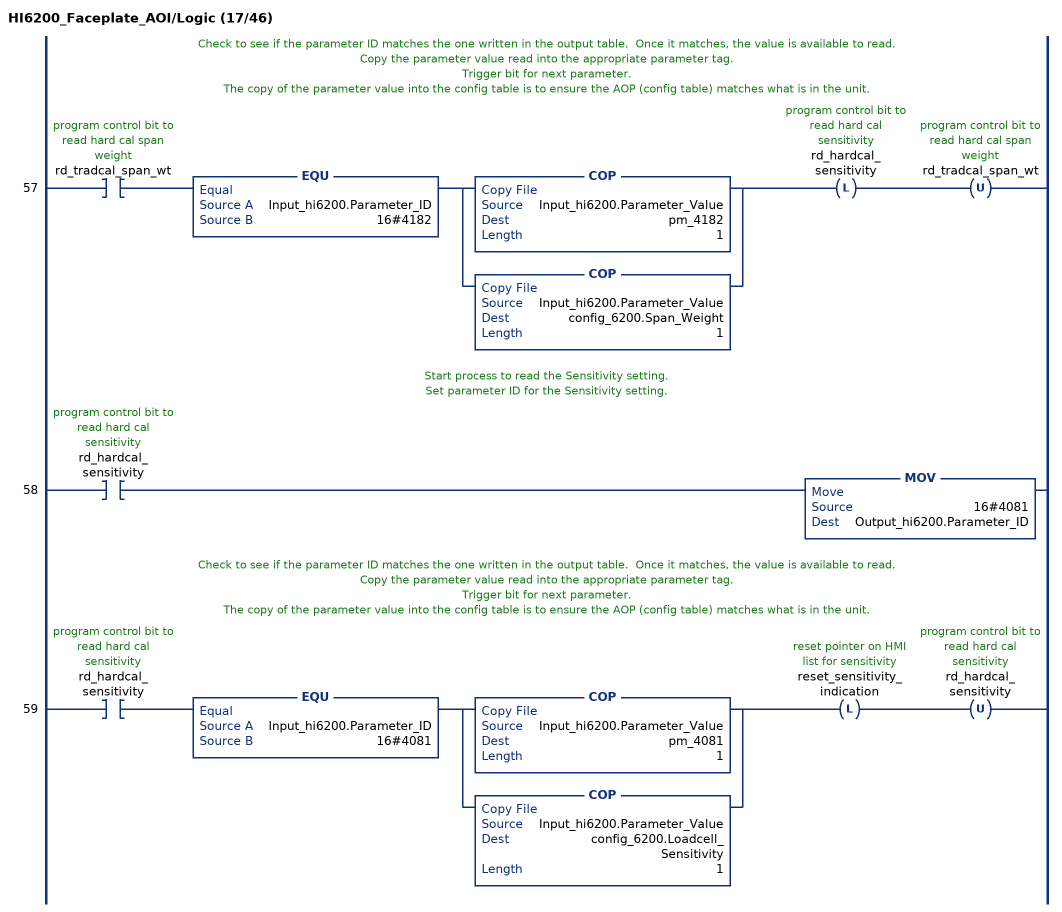
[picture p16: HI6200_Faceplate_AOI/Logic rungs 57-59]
   // Check to see if the parameter ID matches the one written in the output table.  Once it matches, the value is available to read.
   // Copy the parameter value read into the appropriate parameter tag.
   // Trigger bit for next parameter.
   // The copy of the parameter value into the config table is to ensure the AOP (config table) matches what is in the unit.
   57: XIC(rd_tradcal_span_wt)EQU(Input_hi6200.Parameter_ID,16#4182)[COP(Input_hi6200.Parameter_Value,pm_4182,1) ,COP(Input_hi6200.Parameter_Value,config_6200.Span_Weight,1) ]OTL(rd_hardcal_sensitivity)OTU(rd_tradcal_span_wt);
   // Start process to read the Sensitivity setting.
   // Set parameter ID for the Sensitivity setting.
   58: XIC(rd_hardcal_sensitivity)MOV(16#4081,Output_hi6200.Parameter_ID);
   // Check to see if the parameter ID matches the one written in the output table.  Once it matches, the value is available to read.
   // Copy the parameter value read into the appropriate parameter tag.
   // Trigger bit for next parameter.
   // The copy of the parameter value into the config table is to ensure the AOP (config table) matches what is in the unit.
   59: XIC(rd_hardcal_sensitivity)EQU(Input_hi6200.Parameter_ID,16#4081)[COP(Input_hi6200.Parameter_Value,pm_4081,1) ,COP(Input_hi6200.Parameter_Value,config_6200.Loadcell_Sensitivity,1) ]OTL(reset_sensitivity_indication)OTU(rd_hardcal_sensitivity);
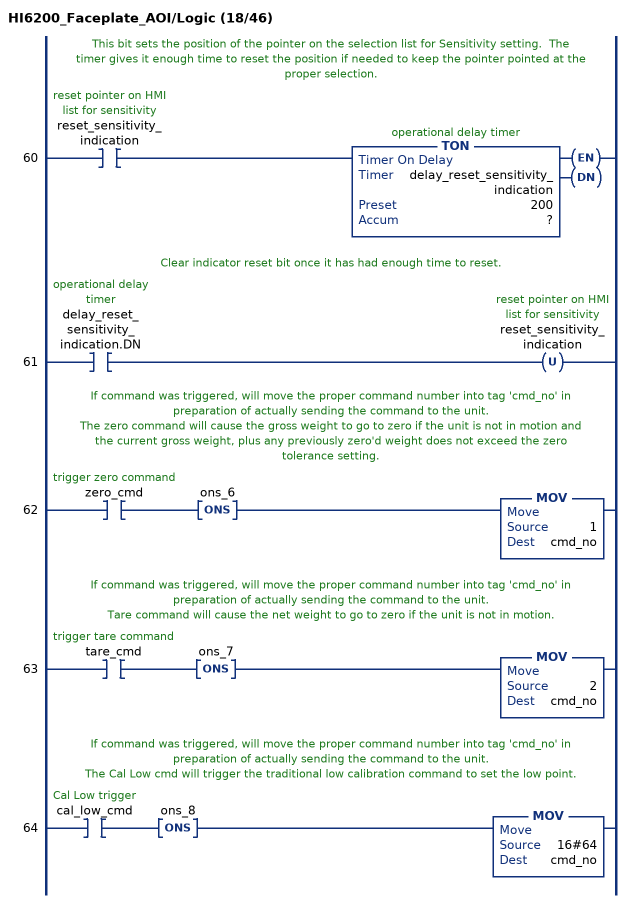
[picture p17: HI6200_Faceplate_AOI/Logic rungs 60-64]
   // This bit sets the position of the pointer on the selection list for Sensitivity setting.  The timer gives it enough time to reset the position if needed to keep the pointer pointed at the proper selection.
   60: XIC(reset_sensitivity_indication)TON(delay_reset_sensitivity_indication,?,?);
   // Clear indicator reset bit once it has had enough time to reset.
   61: XIC(delay_reset_sensitivity_indication.DN)OTU(reset_sensitivity_indication);
   // If command was triggered, will move the proper command number into tag 'cmd_no' in preparation of actually sending the command to the unit.
   // The zero command will cause the gross weight to go to zero if the unit is not in motion and the current gross weight, plus any previously zero'd weight does not exceed the zero tolerance setting.
   62: XIC(zero_cmd)ONS(ons_6)MOV(1,cmd_no);
   // If command was triggered, will move the proper command number into tag 'cmd_no' in preparation of actually sending the command to the unit.
   // Tare command will cause the net weight to go to zero if the unit is not in motion.
   63: XIC(tare_cmd)ONS(ons_7)MOV(2,cmd_no);
   // If command was triggered, will move the proper command number into tag 'cmd_no' in preparation of actually sending the command to the unit.
   // The Cal Low cmd will trigger the traditional low calibration command to set the low point.
   64: XIC(cal_low_cmd)ONS(ons_8)MOV(16#64,cmd_no);
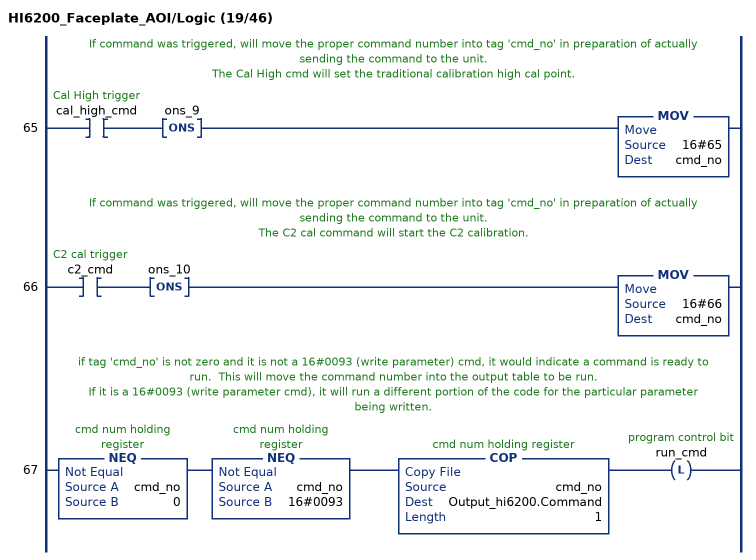
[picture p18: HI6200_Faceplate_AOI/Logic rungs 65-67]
   // If command was triggered, will move the proper command number into tag 'cmd_no' in preparation of actually sending the command to the unit.
   // The Cal High cmd will set the traditional calibration high cal point.
   65: XIC(cal_high_cmd)ONS(ons_9)MOV(16#65,cmd_no);
   // If command was triggered, will move the proper command number into tag 'cmd_no' in preparation of actually sending the command to the unit.
   // The C2 cal command will start the C2 calibration.
   66: XIC(c2_cmd)ONS(ons_10)MOV(16#66,cmd_no);
   // if tag 'cmd_no' is not zero and it is not a 16#0093 (write parameter) cmd, it would indicate a command is ready to run.  This will move the command number into the output table to be run.
   // If it is a 16#0093 (write parameter cmd), it will run a different portion of the code for the particular parameter being written.
   67: NEQ(cmd_no,0)NEQ(cmd_no,16#0093)COP(cmd_no,Output_hi6200.Command,1)OTL(run_cmd);
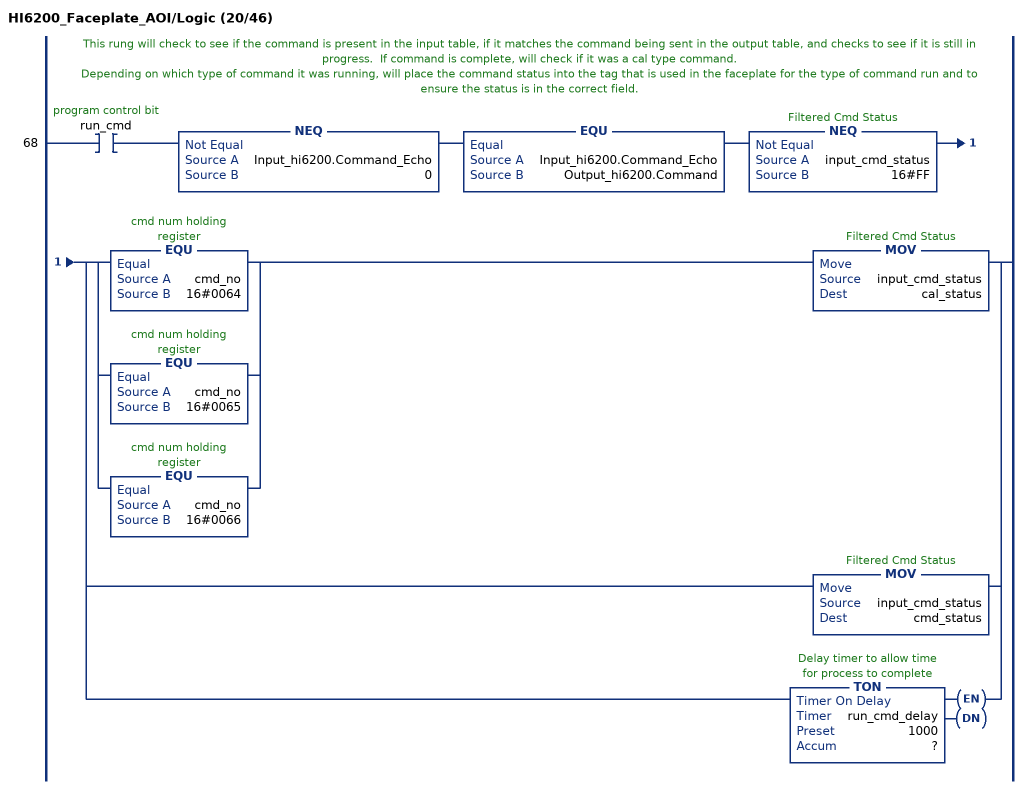
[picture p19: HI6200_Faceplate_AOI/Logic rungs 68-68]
   // This rung will check to see if the command is present in the input table, if it matches the command being sent in the output table, and checks to see if it is still in progress.  If command is complete, will check if it was a cal type command.
   // Depending on which type of command it was running, will place the command status into the tag that is used in the faceplate for the type of command run and to ensure the status is in the correct field.
   68: XIC(run_cmd)NEQ(Input_hi6200.Command_Echo,0)EQU(Input_hi6200.Command_Echo,Output_hi6200.Command)NEQ(input_cmd_status,16#FF)[[EQU(cmd_no,16#0064) ,EQU(cmd_no,16#0065) ,EQU(cmd_no,16#0066) ] MOV(input_cmd_status,cal_status) ,MOV(input_cmd_status,cmd_status) ,TON(run_cmd_delay,?,?) ];
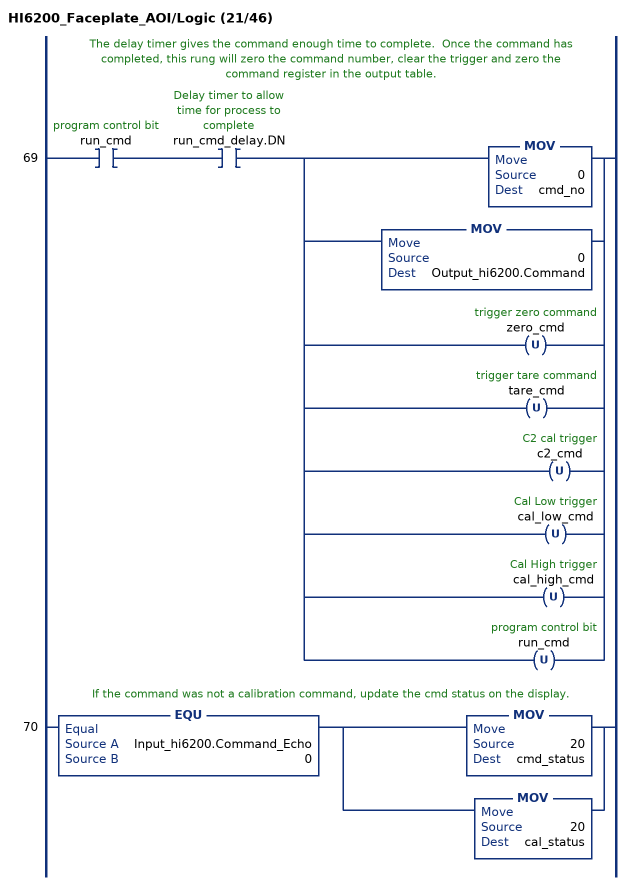
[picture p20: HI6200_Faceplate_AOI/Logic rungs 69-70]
   // The delay timer gives the command enough time to complete.  Once the command has completed, this rung will zero the command number, clear the trigger and zero the command register in the output table.
   69: XIC(run_cmd)XIC(run_cmd_delay.DN)[MOV(0,cmd_no) ,MOV(0,Output_hi6200.Command) ,OTU(zero_cmd) ,OTU(tare_cmd) ,OTU(c2_cmd) ,OTU(cal_low_cmd) ,OTU(cal_high_cmd) ,OTU(run_cmd) ];
   // If the command was not a calibration command, update the cmd status on the display.
   70: EQU(Input_hi6200.Command_Echo,0)[MOV(20,cmd_status) ,MOV(20,cal_status) ];
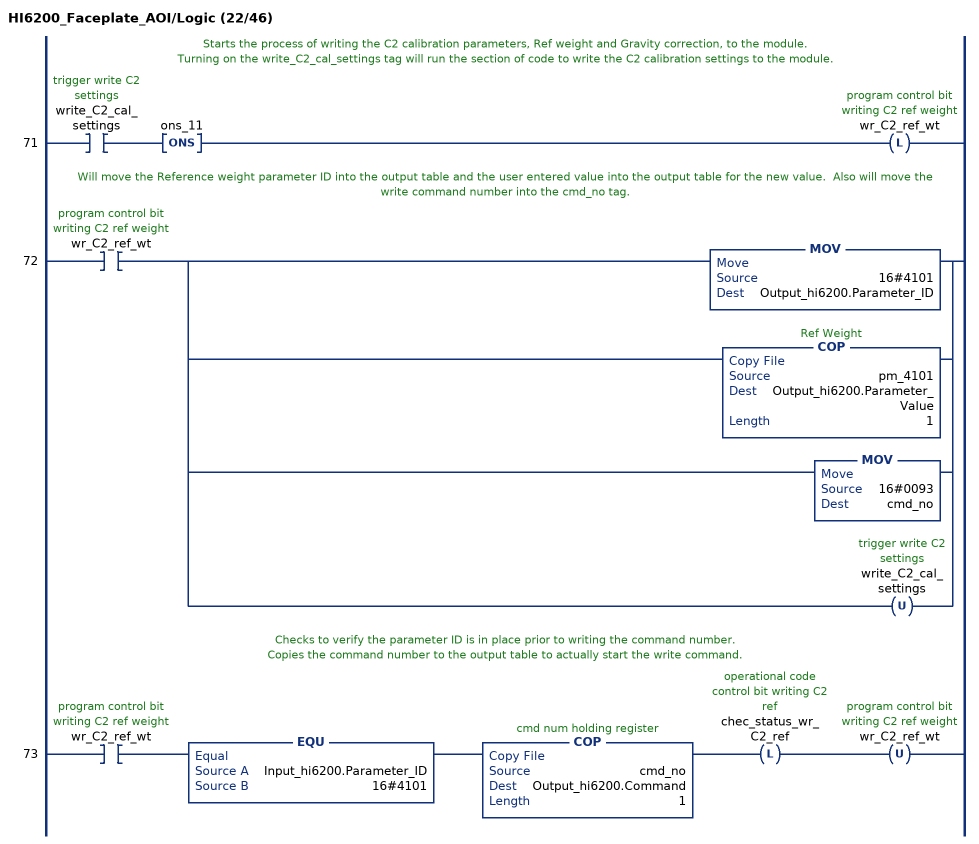
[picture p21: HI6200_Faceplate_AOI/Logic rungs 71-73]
   // Starts the process of writing the C2 calibration parameters, Ref weight and Gravity correction, to the module.
   // Turning on the write_C2_cal_settings tag will run the section of code to write the C2 calibration settings to the module.
   71: XIC(write_C2_cal_settings)ONS(ons_11)OTL(wr_C2_ref_wt);
   // Will move the Reference weight parameter ID into the output table and the user entered value into the output table for the new value.  Also will move the write command number into the cmd_no tag.
   72: XIC(wr_C2_ref_wt)[MOV(16#4101,Output_hi6200.Parameter_ID) ,COP(pm_4101,Output_hi6200.Parameter_Value,1) ,MOV(16#0093,cmd_no) ,OTU(write_C2_cal_settings) ];
   // Checks to verify the parameter ID is in place prior to writing the command number.
   // Copies the command number to the output table to actually start the write command.
   73: XIC(wr_C2_ref_wt)EQU(Input_hi6200.Parameter_ID,16#4101)COP(cmd_no,Output_hi6200.Command,1)OTL(chec_status_wr_C2_ref)OTU(wr_C2_ref_wt);
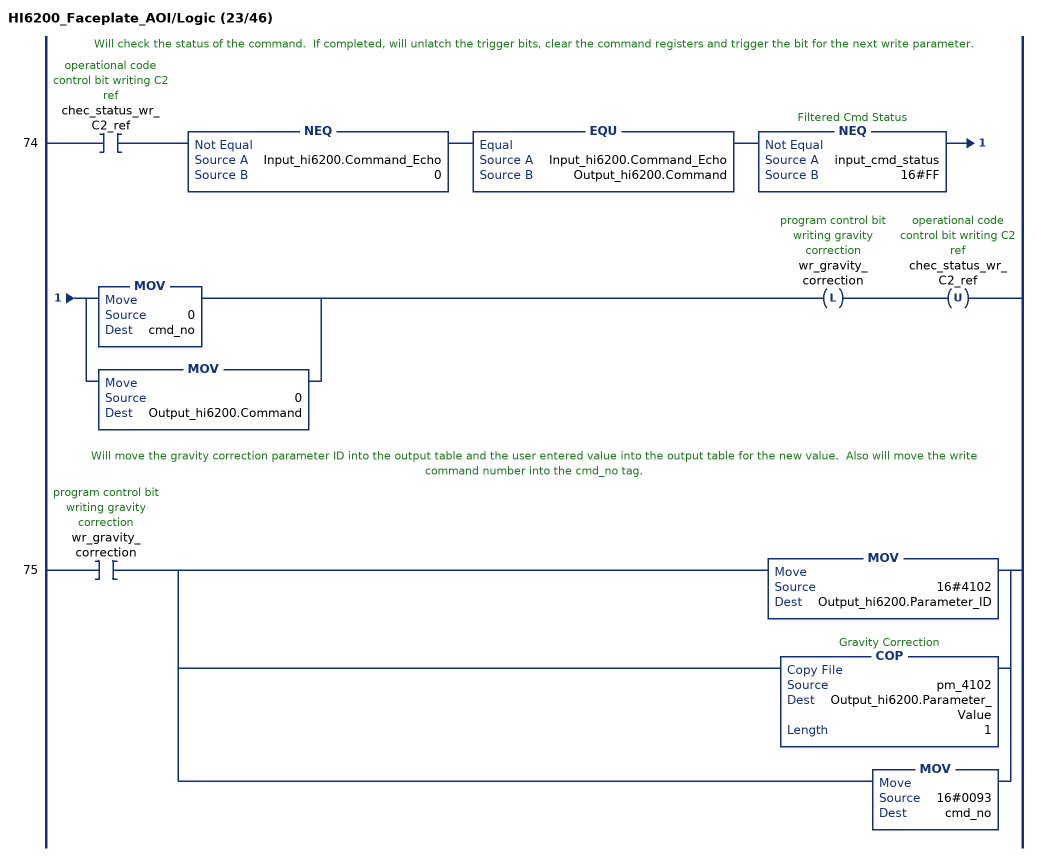
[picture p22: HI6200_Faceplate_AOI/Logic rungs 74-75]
   // Will check the status of the command.  If completed, will unlatch the trigger bits, clear the command registers and trigger the bit for the next write parameter.
   74: XIC(chec_status_wr_C2_ref)NEQ(Input_hi6200.Command_Echo,0)EQU(Input_hi6200.Command_Echo,Output_hi6200.Command)NEQ(input_cmd_status,16#FF)[MOV(0,cmd_no) ,MOV(0,Output_hi6200.Command) ]OTL(wr_gravity_correction)OTU(chec_status_wr_C2_ref);
   // Will move the gravity correction parameter ID into the output table and the user entered value into the output table for the new value.  Also will move the write command number into the cmd_no tag.
   75: XIC(wr_gravity_correction)[MOV(16#4102,Output_hi6200.Parameter_ID) ,COP(pm_4102,Output_hi6200.Parameter_Value,1) ,MOV(16#0093,cmd_no) ];
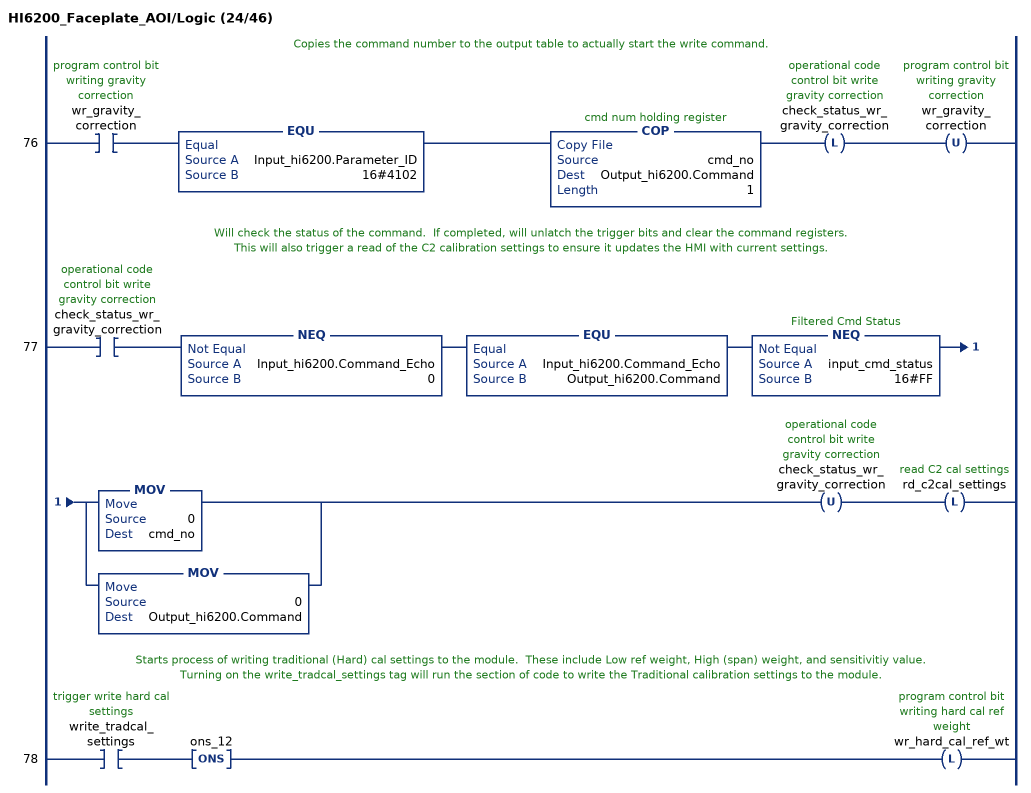
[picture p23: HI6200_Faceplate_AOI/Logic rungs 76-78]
   // Copies the command number to the output table to actually start the write command.
   76: XIC(wr_gravity_correction)EQU(Input_hi6200.Parameter_ID,16#4102)COP(cmd_no,Output_hi6200.Command,1)OTL(check_status_wr_gravity_correction)OTU(wr_gravity_correction);
   // Will check the status of the command.  If completed, will unlatch the trigger bits and clear the command registers.
   // This will also trigger a read of the C2 calibration settings to ensure it updates the HMI with current settings.
   77: XIC(check_status_wr_gravity_correction)NEQ(Input_hi6200.Command_Echo,0)EQU(Input_hi6200.Command_Echo,Output_hi6200.Command)NEQ(input_cmd_status,16#FF)[MOV(0,cmd_no) ,MOV(0,Output_hi6200.Command) ]OTU(check_status_wr_gravity_correction)OTL(rd_c2cal_settings);
   // Starts process of writing traditional (Hard) cal settings to the module.  These include Low ref weight, High (span) weight, and sensitivitiy value.
   // Turning on the write_tradcal_settings tag will run the section of code to write the Traditional calibration settings to the module.
   78: XIC(write_tradcal_settings)ONS(ons_12)OTL(wr_hard_cal_ref_wt);
